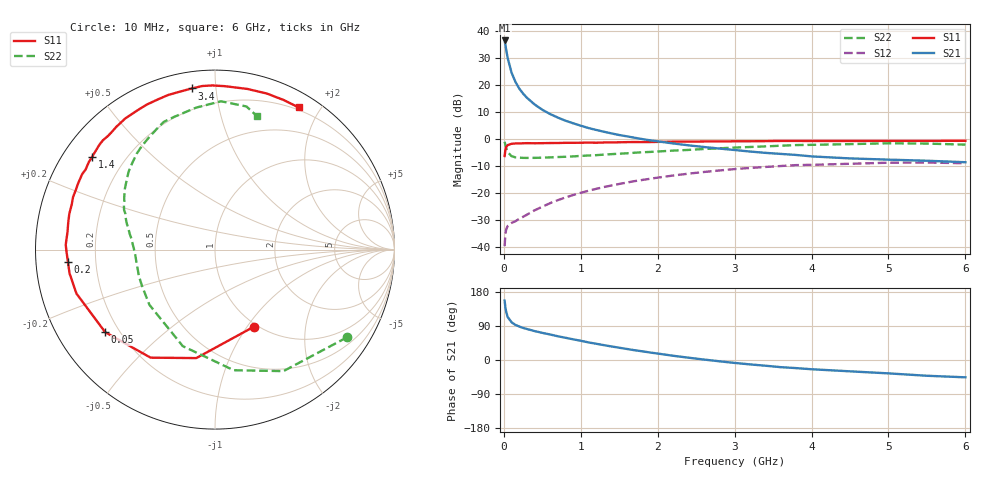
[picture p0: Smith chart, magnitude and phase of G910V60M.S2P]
! SIEMENS Small Signal Semiconductors
! BFG235
! Si NPN RF Bipolar Junction Transistor in SOT223
! VCE = 10 V  IC = 60 mA
! Common Emitter S-Parameters:  July  1994
# GHz  S  MA  R  50
!  f  S11  S21  S12  S22
! GHz  MAG  ANG  MAG  ANG  MAG  ANG  MAG  ANG
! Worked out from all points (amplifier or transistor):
!   40 points, 10 MHz to 6 GHz, reference 50 ohm
!   highest |S21| = 36.4 dB at 10 MHz (marker M1)
!   |S21| within 3 dB of that: start of sweep to 28.01 MHz
!   unconditionally stable (mu >= 1): 499.6 MHz to 1.387 GHz
!   at 200 MHz: K = 0.69, MSG = 24.1 dB, |S12| = -29.6 dB
!   at 1.5 GHz: K = 0.98, MSG = 9.1 dB, |S12| = -16.7 dB
!   at 6 GHz: K = 0.92, MSG = 0.2 dB, |S12| = -9.0 dB
!   S11 on the Smith chart (normalised r, x): 10 MHz: 0.96, -1.07; 50 MHz: 0.15, -0.33; 200 MHz: 0.10, -0.04; 1.4 GHz: 0.09, +0.33; 3.4 GHz: 0.09, +0.86; 6 GHz: 0.17, +1.74
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0.01  0.4813 -63.5  66.25 156.8  0.0103 68.0  0.8831 -33.6
0.02  0.6134 -99.8  54.96 139.4  0.0169 54.1  0.7771 -60.6
0.03  0.7009 -120.8  45.09 127.4  0.021 44.2  0.6801 -81.2
0.05  0.7656 -143.1  31.18 113.5  0.0244 34.7  0.5668 -108.5
0.1  0.8099 -162.4  16.86 99.6  0.0277 31.7  0.4777 -139.9
0.15  0.8211 -170.7  11.38 92.7  0.0298 35.5  0.4542 -153.7
0.2  0.8223 -175.3  8.542 88.4  0.033 39.3  0.4486 -161.2
0.25  0.8271 -179.0  6.882 84.7  0.036 43.2  0.444 -166.1
0.3  0.8321 178.1  5.753 81.8  0.0394 46.2  0.4437 -169.9
0.4  0.8276 173.3  4.326 76.3  0.0475 51.0  0.4442 -174.8
0.5  0.8317 169.4  3.454 71.6  0.0554 53.8  0.4482 -178.4
0.6  0.8359 166.1  2.882 67.4  0.0643 55.4  0.4535 178.6
0.7  0.837 162.4  2.48 62.7  0.0731 56.7  0.4602 176.0
0.9  0.8437 156.8  1.942 54.6  0.091 56.4  0.4728 171.8
1.1  0.8512 150.4  1.586 46.4  0.1093 55.0  0.4912 167.6
1.4  0.8577 143.1  1.259 35.7  0.1369 51.7  0.5208 161.9
2.2  0.8855 124.3  0.821 11.2  0.2091 38.9  0.6053 146.1
3.2  0.9015 102.5  0.582 -11.6  0.2888 19.3  0.7063 125.3
3.4  0.907 98.2  0.55 -15.1  0.3013 15.1  0.7247 120.6
4.5  0.9131 78.6  0.434 -29.9  0.3453 -6.8  0.7981 97.5
5.5  0.917 65.3  0.393 -41.6  0.3643 -25.7  0.8165 77.6
6  0.9191 59.5  0.369 -45.7  0.3532 -32.5  0.7807 72.7
